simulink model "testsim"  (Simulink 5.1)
settings: Solver=ode23tb  StartTime=0  StopTime=1200  MaxStep=.1  RelTol=1e-3
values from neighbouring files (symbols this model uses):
  c0 = [0 0 1]    [runcases.m]
  c1 = [0 1 1]    [runcases.m]
  f0 = [0 0 0]    [runcases.m]
  f1 = [0 1 2]    [runcases.m]
  l0 = [0 0 0]    [runcases.m]
  l1 = [0 0 1]    [runcases.m]
  t0 = [1 1 1]    [runcases.m]
  t1 = [1 0.95 0.95]    [runcases.m]
  tc = [0;140;0]    [runcases.m]
  tflt = [0;110;100]    [runcases.m]
  tl = [0;0;140]    [runcases.m]
  tt = [0;140;140]    [runcases.m]
undefined symbols (not defined in the file or in its folder): primarycontrolled

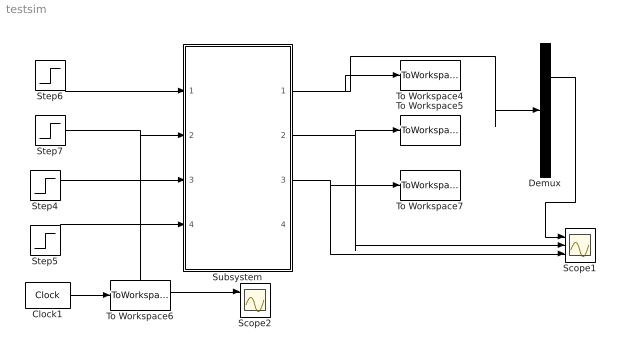
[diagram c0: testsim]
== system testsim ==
  Clock1 : Clock
  Demux : Demux  Outputs=[3 2 3]
  Scope1 : Scope  NumInputPorts=3
  Scope2 : Scope  NumInputPorts=3
  Step4 : Step  Time=tt  Before=t0  After=t1  SampleTime=0
  Step5 : Step  Time=tflt  Before=f0  After=f1  SampleTime=0
  Step6 : Step  Time=tc  Before=c0  After=c1  SampleTime=0
  Step7 : Step  Time=tl  Before=l0  After=l1  SampleTime=0
  Subsystem : Subsystem
  To Workspace4 : ToWorkspace  VariableName=V  SampleTime=-1  SaveFormat=Array
  To Workspace5 : ToWorkspace  VariableName=Efd  SampleTime=-1  SaveFormat=Array
  To Workspace6 : ToWorkspace  VariableName=t  SampleTime=-1  SaveFormat=Array
  To Workspace7 : ToWorkspace  VariableName=tappos  SampleTime=-1  SaveFormat=Array
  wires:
  Subsystem/1(V) -> To Workspace4/1, Demux/1
  Clock1/1 -> To Workspace6/1
  Step5/1 -> Subsystem/4(Faulted)
  Step7/1 -> Subsystem/2(LoadStep), Scope2/1
  Step4/1 -> Subsystem/3(TapVref)
  Subsystem/3(Tappos) -> To Workspace7/1, Scope1/3
  Subsystem/2(Efd) -> To Workspace5/1, Scope1/2
  Demux/1 -> Scope1/1
  Step6/1 -> Subsystem/1(CapStep)

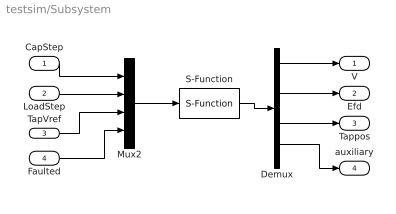
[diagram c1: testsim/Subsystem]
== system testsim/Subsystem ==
  CapStep : Inport
  LoadStep : Inport  Port=2
  TapVref : Inport  Port=3
  Faulted : Inport  Port=4
  Demux : Demux  Outputs="[8  2 3  14]"
  Mux2 : Mux  Inputs=[3 3 3 3]
  S-Function : S-Function  FunctionName=primarycontrolledd  Parameters=primarycontrolled.p,primarycontrolled.x0
  V : Outport
  Efd : Outport  Port=2
  Tappos : Outport  Port=3
  auxiliary : Outport  Port=4
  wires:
  CapStep/1 -> Mux2/1
  LoadStep/1 -> Mux2/2
  TapVref/1 -> Mux2/3
  Faulted/1 -> Mux2/4
  Mux2/1 -> S-Function/1
  S-Function/1 -> Demux/1
  Demux/1 -> V/1
  Demux/2 -> Efd/1
  Demux/4 -> auxiliary/1
  Demux/3 -> Tappos/1
